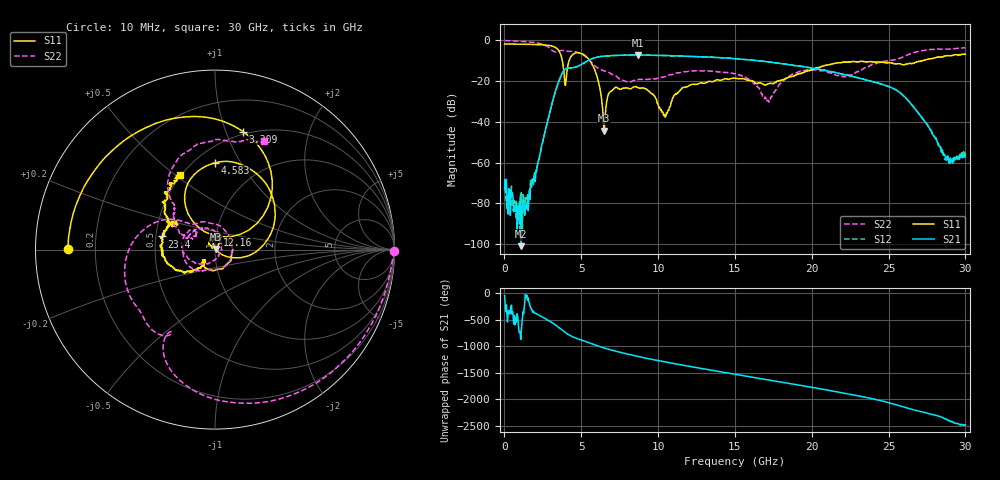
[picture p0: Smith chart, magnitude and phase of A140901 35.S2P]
!  2-Port S-parameters saved by WinCal
! VAR MeasName=S-Parameters (CALIBRATED_DATA) read from VNA (N5244A)
! VAR MeasDate=11/3/2014 9:33:20 AM
! VAR NAME=A140901 35
! VAR FILENAME=A140901 35.S2P
! VAR DATE=11/3/2014 9:33:20 AM
! VAR PHYS_PORTS=1,2
# Hz S RI R 50
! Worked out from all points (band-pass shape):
!   801 points, 10 MHz to 30 GHz, reference 50 ohm
!   highest |S21| = -7.13 dB at 8.67 GHz (marker M1); lowest = -101.1 dB at 1.097 GHz (marker M2)
!   |S21| within 3 dB of the highest: 5.397 GHz to 16.7 GHz (11.31 GHz wide, 102 % of centre)
!   lowest |S11| = -44.4 dB at 6.495 GHz (marker M3), VSWR 1.01, Z = 50.5 + j0.39 ohm
!   |S11| at or under -10 dB: 3.766 GHz to 4.204 GHz (437.7 MHz wide, 11 % of centre); 5.563 GHz to 27.23 GHz (21.67 GHz wide, 132 % of centre)
!   |S22| runs from -30.3 to 0.0 dB; largest |S21 - S12| = 0.0039
!   S11 on the Smith chart (normalised r, x): 10 MHz: 0.10, +0.00; 3.309 GHz: 0.47, +1.15; 4.583 GHz: 0.62, +0.78; 12.16 GHz: 1.01, +0.17; 23.4 GHz: 0.54, +0.09; 30 GHz: 0.49, +0.52
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1e7  -0.8176 0.0029  0.00016 -0.000166  -0.000213 -2.78e-05  0.9981 -0.00732
1.097138e9  -0.7308 0.3469  8.06e-06 3.55e-06  -3.18e-05 -0.00018  0.7237 -0.615
1.5095e9  -0.6521 0.4651  -0.000106 -0.000121  1.19e-05 -7.33e-05  0.5198 -0.7684
3.3089e9  0.1561 0.6577  -0.0316 0.0452  -0.0318 0.045  -0.2437 -0.4585
3.983675e9  -0.0152 0.0808  0.183 -0.0805  0.1832 -0.0802  -0.3982 -0.3791
4.583475e9  -0.000863 0.4833  -0.103 -0.1924  -0.1028 -0.1925  -0.4992 -0.1788
5.033325e9  0.264 0.3919  -0.2517 -0.0618  -0.2514 -0.0625  -0.4608 0.0366
5.895538e9  0.1775 -0.0373  -0.0904 0.3653  -0.0915 0.366  -0.1759 0.1566
6.495338e9  0.00464 0.00386  0.2814 0.2992  0.2815 0.3  -0.1012 0.1452
7.095138e9  -0.00136 0.0628  0.4251 -0.0192  0.4252 -0.0189  0.00311 0.1411
8.669612e9  0.00658 0.0696  -0.1647 -0.4081  -0.1646 -0.4077  0.0562 -0.0918
1.001916e10  0.0166 0.0187  -0.4212 0.0924  -0.4201 0.0921  -0.0404 -0.1134
1.05065e10  -0.00797 0.0116  -0.3286 0.2722  -0.3285 0.2714  -0.0618 -0.116
1.215595e10  0.0136 0.081  0.242 0.3232  0.2401 0.3236  -0.1626 -0.0706
1.5005e10  -0.021 -0.1152  -0.000937 -0.3557  -0.000774 -0.3567  -0.0989 0.1134
1.714179e10  -0.0594 -0.0601  -0.2858 0.0838  -0.2863 0.0834  0.0324 -0.0107
2.002832e10  -0.1482 -0.1201  0.1951 0.0751  0.1957 0.0761  -0.177 0.0603
2.34022e10  -0.2959 0.0734  -0.1039 -0.0376  -0.104 -0.0377  -0.1907 0.0849
2.501416e10  -0.2331 0.1535  -0.00278 0.0734  -0.00312 0.0733  -0.2244 0.2283
2.681356e10  -0.2496 0.1493  0.0105 -0.0156  0.0104 -0.0156  -0.2283 0.4704
2.876291e10  -0.2709 0.3175  -0.000761 0.00085  -0.000806 0.000854  0.1014 0.6016
3e10  -0.1974 0.4159  0.00146 0.000772  0.00119 0.000303  0.2702 0.6033
